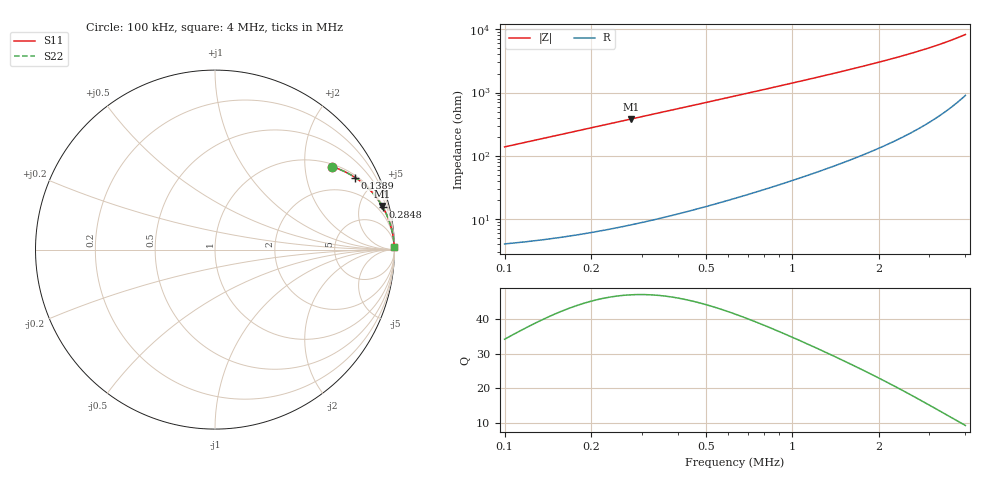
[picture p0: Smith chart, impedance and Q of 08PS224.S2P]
! Coilcraft 0805PS-224 Power Chip Inductor
! 5 February 2003
# MHZ S MA R 50
!Freq  MagS11  AngS11  MagS21  AngS21  MagS12  AngS12  MagS22  AngS22
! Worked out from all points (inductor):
!   402 points, 100 kHz to 4 MHz, reference 50 ohm
!   read as one part in series: L = 220 uH near 119.5 kHz
!   highest Q = 47.1 at 275.1 kHz (marker M1), where L = 220 uH
!   S11 on the Smith chart (normalised r, x): 100 kHz: 1.08, +2.76; 138.9 kHz: 1.10, +3.84; 284.8 kHz: 1.17, +7.89; 4 MHz: open
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0.1  0.7993 35.3  0.5779 -53.0  0.5779 -53.0  0.7993 35.3
0.119452  0.8456 30.8  0.5118 -57.7  0.5118 -57.7  0.8456 30.8
0.138904  0.8782 27.2  0.4571 -61.4  0.4571 -61.4  0.8782 27.2
0.168082  0.911 23.1  0.3918 -65.6  0.3918 -65.6  0.911 23.1
0.19726  0.9323 20.0  0.3416 -68.8  0.3416 -68.8  0.9323 20.0
0.236164  0.9505 16.9  0.2908 -71.9  0.2908 -71.9  0.9505 16.9
0.275068  0.9622 14.6  0.2526 -74.2  0.2526 -74.2  0.9622 14.6
0.284794  0.9645 14.2  0.2446 -74.6  0.2446 -74.6  0.9645 14.2
0.323698  0.9717 12.5  0.2167 -76.3  0.2167 -76.3  0.9717 12.5
0.372328  0.9778 10.9  0.1894 -77.9  0.1894 -77.9  0.9778 10.9
0.479314  0.9857 8.5  0.1481 -80.2  0.1481 -80.2  0.9857 8.5
0.605752  0.9903 6.7  0.1174 -81.9  0.1174 -81.9  0.9903 6.7
0.751642  0.9931 5.4  0.09446 -83.1  0.09446 -83.1  0.9931 5.4
0.887806  0.9946 4.6  0.07972 -83.9  0.07972 -83.9  0.9946 4.6
1.043422  0.9957 3.9  0.06747 -84.5  0.06747 -84.5  0.9957 3.9
1.21849  0.9965 3.3  0.05734 -84.9  0.05734 -84.9  0.9965 3.3
1.403284  0.9971 2.8  0.04929 -85.2  0.04929 -85.2  0.9971 2.8
1.70479  0.9977 2.3  0.03977 -85.5  0.03977 -85.5  0.9977 2.3
2.054926  0.9981 1.8  0.03204 -85.6  0.03204 -85.6  0.9981 1.8
2.706568  0.9984 1.3  0.0226 -85.4  0.0226 -85.4  0.9984 1.3
3.35821  0.9986 0.9  0.01645 -84.6  0.01645 -84.6  0.9986 0.9
4  0.9986 0.7  0.01206 -83.1  0.01206 -83.1  0.9986 0.7
